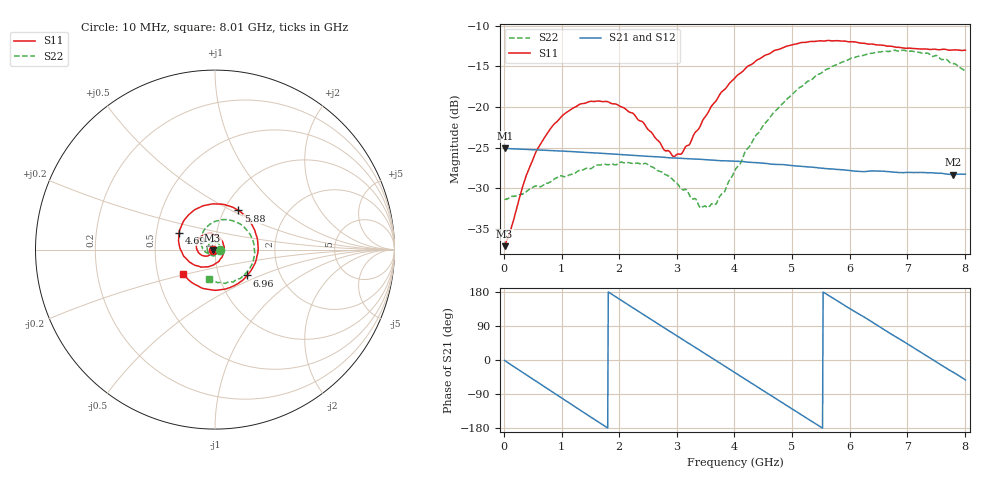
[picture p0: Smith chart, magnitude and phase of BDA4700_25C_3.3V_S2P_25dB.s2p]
!Agilent Technologies,E5071B,MY42404982,A.09.10
!Date: Mon Oct 20 18:13:34 2025
!Data & Calibration Information:
!Freq	S11:SOLT2(ON)	S21:SOLT2(ON)	S12:SOLT2(ON)	S22:SOLT2(ON)
# Hz S RI R 50
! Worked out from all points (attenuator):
!   801 points, 10 MHz to 8.01 GHz, reference 50 ohm
!   highest |S21| = -25.06 dB at 20 MHz (marker M1); lowest = -28.3 dB at 7.8 GHz (marker M2)
!   lowest |S11| = -37.1 dB at 10 MHz (marker M3), VSWR 1.03, Z = 48.6 - j0.13 ohm
!   |S11| at or under -10 dB: start of sweep to end of sweep
!   |S22| runs from -32.4 to -13.0 dB; largest |S21 - S12| = 0.00062
!   S11 on the Smith chart (normalised r, x): 10 MHz: 0.97, -0.00; 4.69 GHz: 0.66, +0.13; 5.88 GHz: 1.16, +0.54; 6.96 GHz: 1.36, -0.41; 8.01 GHz: 0.67, -0.19
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1e7  -0.0139 -0.00133  0.0558 -0.00117  0.0558 -0.00121  0.0271 -0.000808
2e7  -0.0143 -0.00214  0.0558 -0.00212  0.0557 -0.00223  0.027 -0.00106
3.6e8  -0.0245 -0.0259  0.0441 -0.0327  0.0441 -0.0328  0.0227 -0.019
5.8e8  -0.0418 -0.0359  0.0284 -0.0466  0.0284 -0.0466  0.0144 -0.0292
1e9  -0.084 -0.0244  -0.0097 -0.0527  -0.00967 -0.0528  -0.0146 -0.0348
1.35e9  -0.104 0.0133  -0.0374 -0.0372  -0.0374 -0.0373  -0.0366 -0.0182
1.97e9  -0.0588 0.085  -0.0492 0.0143  -0.0492 0.0143  -0.0347 0.028
2.68e9  0.0414 0.0461  -0.00412 0.0492  -0.00413 0.0492  0.0131 0.0383
2.93e9  0.0498 0.00274  0.0161 0.0459  0.0161 0.0458  0.0253 0.0253
3.06e9  0.0466 -0.0214  0.0257 0.0411  0.0253 0.0413  0.028 0.0154
3.43e9  0.000376 -0.0799  0.0441 0.0182  0.0441 0.0183  0.0201 -0.0131
3.69e9  -0.0542 -0.0962  0.0469 -0.00205  0.047 -0.00217  0.00146 -0.0255
4.01e9  -0.1299 -0.0769  0.0389 -0.0256  0.0388 -0.0255  -0.0312 -0.026
4.69e9  -0.2008 0.095  -0.00713 -0.0439  -0.00697 -0.0439  -0.0799 0.0481
5.35e9  -0.0549 0.2466  -0.0408 -0.0128  -0.0406 -0.013  -0.0159 0.1473
5.88e9  0.1307 0.2181  -0.0346 0.0223  -0.0346 0.0221  0.1023 0.1593
6.27e9  0.2217 0.1069  -0.015 0.0372  -0.0143 0.0373  0.1831 0.1017
6.68e9  0.2314 -0.0496  0.0121 0.0382  0.0122 0.0382  0.2198 0.000506
6.96e9  0.1788 -0.1439  0.0272 0.0288  0.0273 0.0286  0.2095 -0.0754
7.39e9  0.0332 -0.2234  0.0393 0.00401  0.0392 0.00394  0.1333 -0.1627
7.8e9  -0.1219 -0.1886  0.0324 -0.0206  0.0324 -0.0209  0.0196 -0.1836
8.01e9  -0.1796 -0.1335  0.0234 -0.0307  0.0236 -0.0306  -0.0307 -0.1633
